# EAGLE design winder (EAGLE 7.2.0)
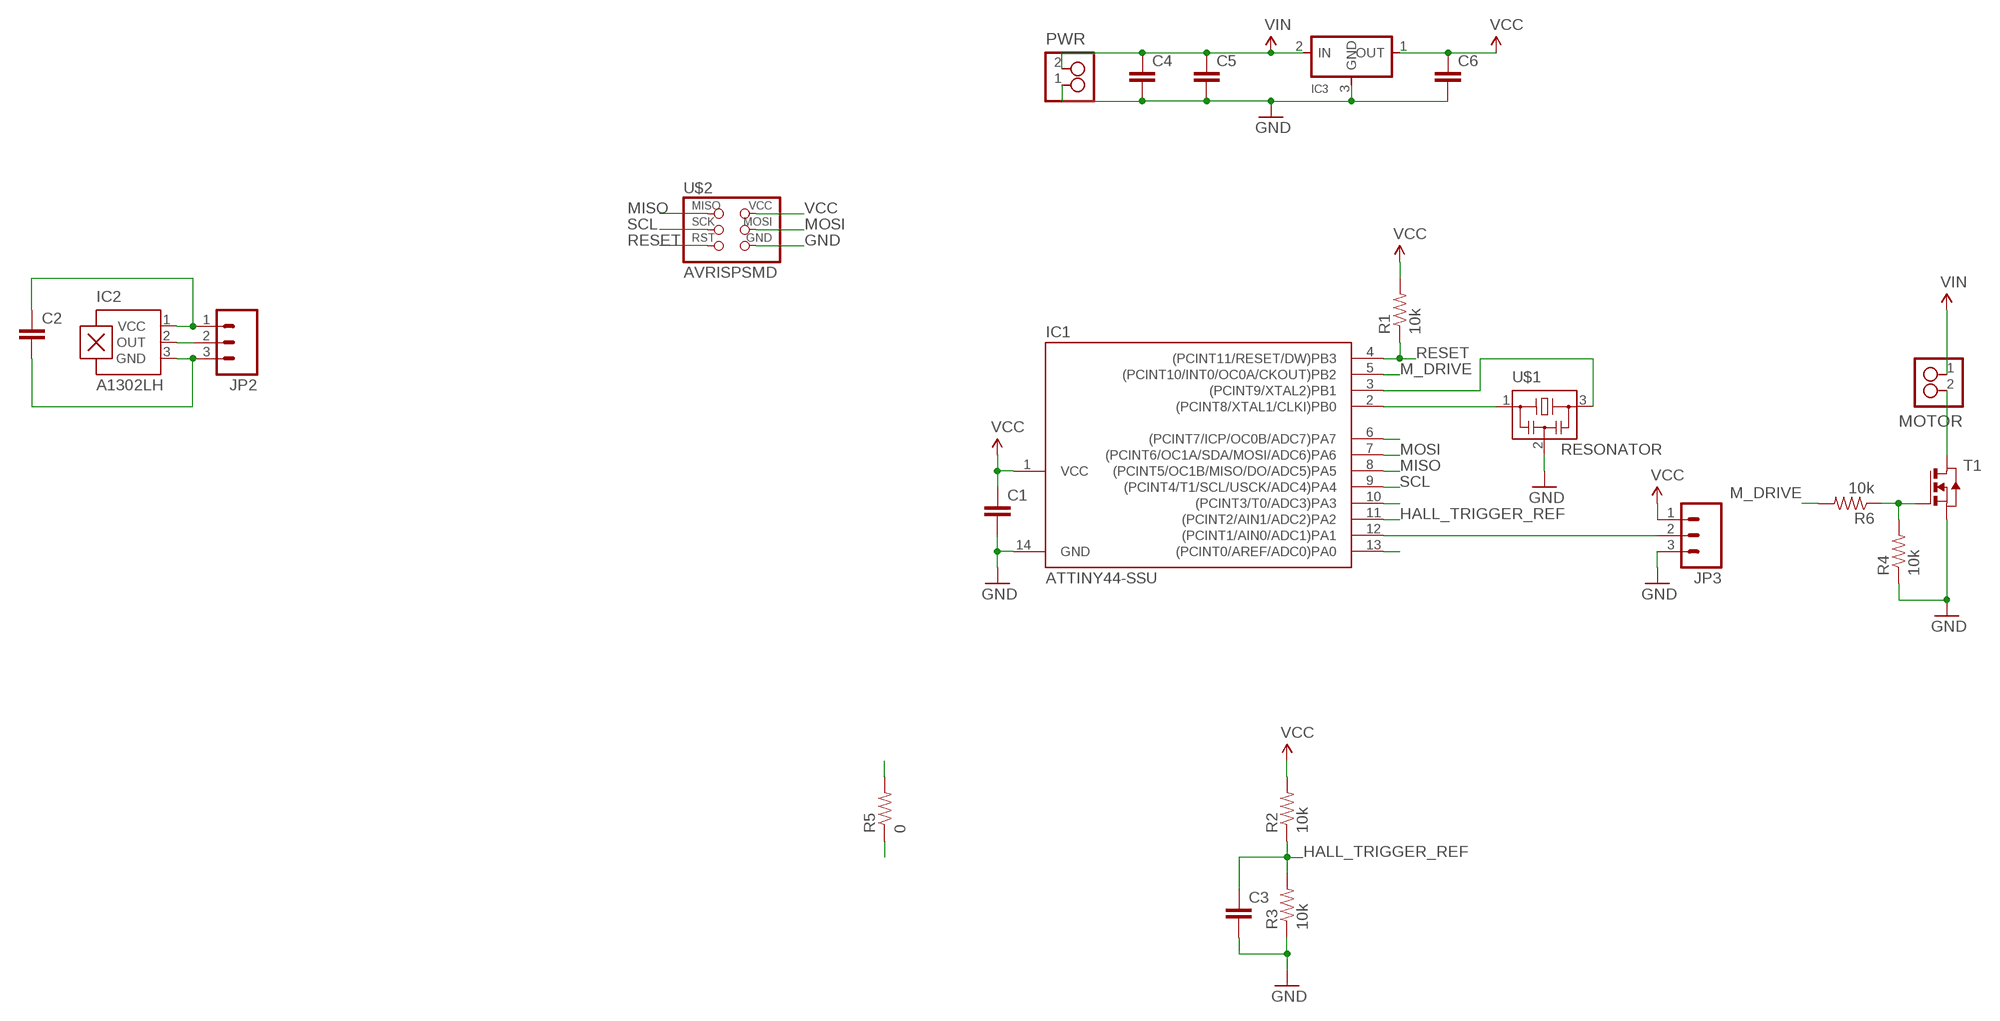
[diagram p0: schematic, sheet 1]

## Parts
C1  CAP1206  [1206]
C2  CAP1206  [1206]
C3  CAP1206  [1206]
C4  CAP1206  [1206]
C5  CAP1206  [1206]
C6  CAP1206  [1206]
IC1  ATTINY44-SSU  [SOIC14]
IC2  A1302LH  [SOT23-W]
IC3  REGULATORSOT23  [SOT23]
JP2  M03SMD_RA_MALE  [1X03_SMD_RA_MALE]
JP3  M03SMD_RA_MALE  [1X03_SMD_RA_MALE]
MOTOR  2_PIN_HEADERSCREW  [SCREW_2]
PWR  2_PIN_HEADERSCREW  [SCREW_2]
R1  10k  RESISTOR1206  [1206]
R2  10k  RESISTOR1206  [1206]
R3  10k  RESISTOR1206  [1206]
R4  10k  RESISTOR1206  [1206]
R5  0  RESISTOR1206  [1206]
R6  10k  RESISTOR1206  [1206]
T1  NMOSFETSOT23  [SOT-23]
U$1  RESONATOR  [EFOBM]
U$2  AVRISPSMD  [2X03SMD]

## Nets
GATE: R4.2 R6.1 T1.3(G)
GND: C1.2 C3.2 C4.2 C5.2 C6.2 IC1.14(GND) IC3.3(GND) JP3.3 PWR.1 R3.1 R4.1 T1.2(S) U$1.2 U$2.6(GND)
HALL_TRIGGER_REF: C3.1 IC1.11((PCINT2/AIN1/ADC2)PA2) R2.1 R3.2
M_DRIVE: IC1.5((PCINT10/INT0/OC0A/CKOUT)PB2) R6.2
MISO: IC1.8((PCINT5/OC1B/MISO/DO/ADC5)PA5) U$2.1(MISO)
MOSI: IC1.7((PCINT6/OC1A/SDA/MOSI/ADC6)PA6) U$2.4(MOSI)
N$1: C2.1 IC2.1(VCC) JP2.1
N$2: IC2.2(OUT) JP2.2
N$3: C2.2 IC2.3(GND) JP2.3
N$4: MOTOR.2 T1.1(D)
N$6: IC1.3((PCINT9/XTAL2)PB1) U$1.3
N$7: IC1.2((PCINT8/XTAL1/CLKI)PB0) U$1.1
N$8: IC1.6((PCINT7/ICP/OC0B/ADC7)PA7)
N$12: IC1.10((PCINT3/T0/ADC3)PA3)
N$14: IC1.12((PCINT1/AIN0/ADC1)PA1) JP3.2
N$15: IC1.13((PCINT0/AREF/ADC0)PA0)
RESET: IC1.4((PCINT11/RESET/DW)PB3) R1.1 U$2.5(RST)
SCL: IC1.9((PCINT4/T1/SCL/USCK/ADC4)PA4) U$2.3(SCK)
VCC: C1.1 C6.1 IC1.1(VCC) IC3.1(OUT) JP3.1 R1.2 R2.2 R5.1 R5.2 U$2.2(VCC)
VIN: C4.1 C5.1 IC3.2(IN) MOTOR.1 PWR.2

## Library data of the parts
C1-C6 = SparkFun-Passives:CAP: Capacitor
IC1 = fab:ATTINY44
IC2 = allegro:A13*?: Linear Hall Effect Sensor ICs Continuous-Time Ratiometric High-Temperature Operation Programmable Linear with Analog Output A1302 -Replacement- UGN3503 Source: http://www.allegromicro.com/en/Products/Part_Numbers/1301/1301.pdf http://www.allegromicro.com/en/Products/Part_Numbers/1321/1321.pdf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; MF: ALLEGRO MICROSYSTEMS, INC.; MPN: A1302ELHLT-T; OC_FARNELL: 1457209; OC_NEWARK: 31K6638
IC3 = fab:REGULATOR
JP2 JP3 = SparkFun-Connectors:M03: Header 3 Standard 3-pin 0.1" header. Use with straight break away headers (SKU : PRT-00116), right angle break away headers (PRT-00553), swiss pins (PRT-00743), machine pins (PRT-00117), and female headers (PRT-00115). Molex polarized connector foot print use with SKU : PRT-08232 with associated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; PROD_ID: CONN-10925
MOTOR PWR = ng:2_PIN_HEADER: 2 SMT pin pads
R1-R6 = SparkFun-Passives:RESISTOR: Resistor
T1 = ng:NMOSFET: MOS FET
U$1 = fab:RESONATOR
U$2 = fab:AVRISP

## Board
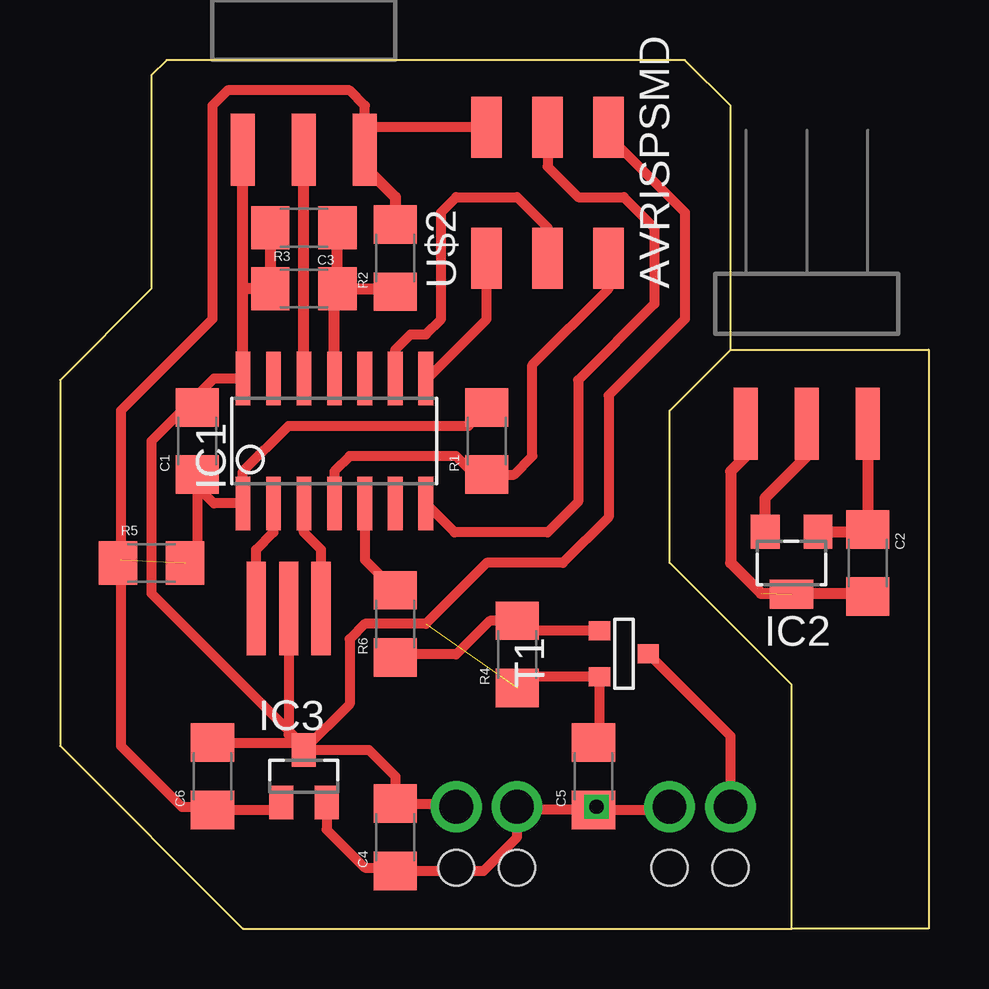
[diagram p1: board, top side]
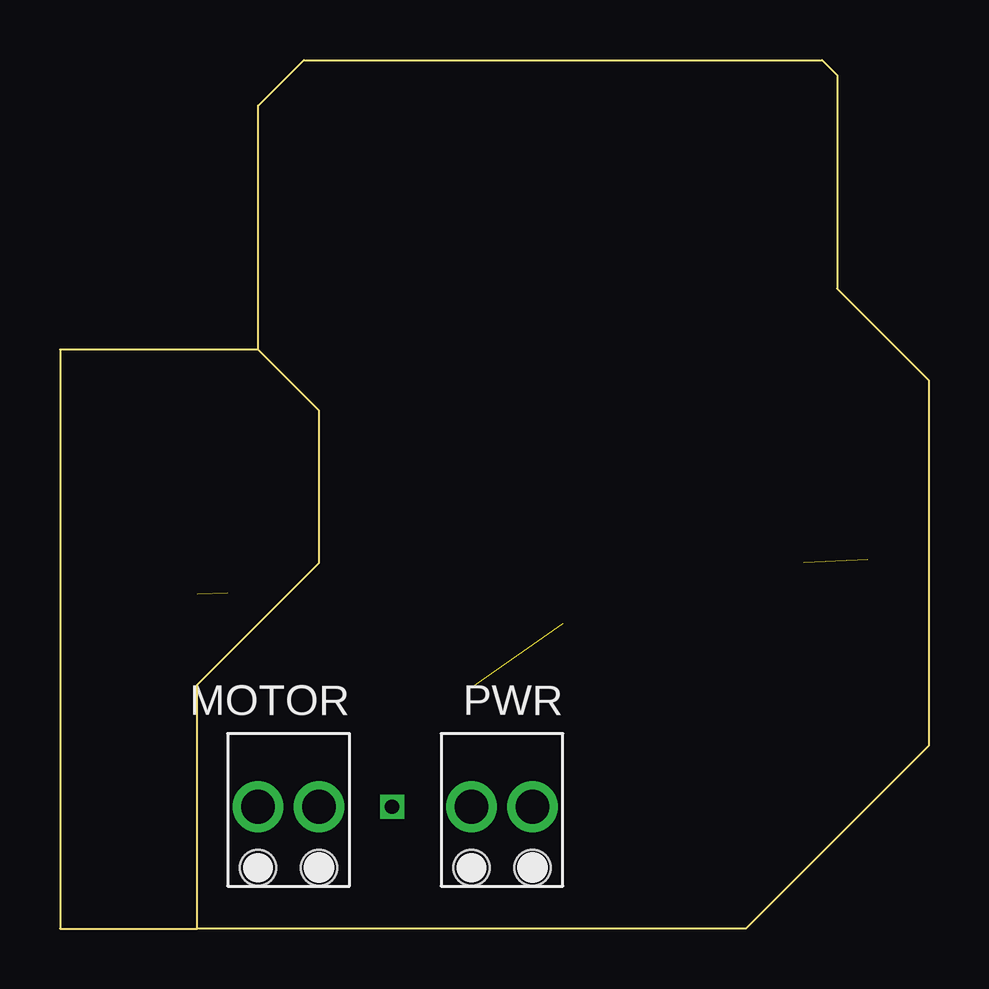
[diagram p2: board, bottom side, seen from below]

Size 36.2 x 36.19 mm. Coordinates in mm from the lower left corner, seen from the top.
Outline: 30.48,0 7.62,0 0,7.62 0,22.86 3.81,26.67 3.81,35.56 4.45,36.19 26.03,36.19 27.94,34.29 27.94,24.13
Outline: 30.48,0 30.48,10.16 25.4,15.24 25.4,21.59 27.94,24.13
Outline: 27.94,24.13 36.2,24.13 36.2,0 30.48,0
Copper layers (1*16): Top 0.035mm / dielectric 1.5mm / Bottom 0.035mm
Design rules "default": minimum track width 10mil, minimum drill 24mil, track to track 8mil, track to pad 8mil, pad to pad 8mil, via to via 8mil, smd to smd 8mil, copper to edge 40mil, drill to drill 8mil, minimum pad ring 10mil, minimum via ring 8mil, stop-mask expansion 4mil, vias tented up to drill 0mil, thermal gap 10mil

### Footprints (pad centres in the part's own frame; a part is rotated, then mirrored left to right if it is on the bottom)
1206 = smd 1.6 x 1.8: 1 -1.4,0; 2 1.4,0
SOIC14 = smd 0.61 x 2.21: 1 -3.81,-2.603; 2 -2.54,-2.603; 3 -1.27,-2.603; 4 0,-2.603; 5 1.27,-2.603; 6 2.54,-2.603; 7 3.81,-2.603; 8 3.81,2.603; 9 2.54,2.603; 10 1.27,2.603; 11 0,2.603; 12 -1.27,2.603; 13 -2.54,2.603; 14 -3.81,2.603
SOT23-W = smd 1.2 x 1.4: 1 -1.1,-1.3; 2 1.1,-1.3 | smd 1.8 x 1.2: 3 0,1.3
SOT23 = smd 1 x 1.4: 1 -0.95,-1.1; 2 0.95,-1.1; 3 0,1.1
1X03_SMD_RA_MALE = smd 1 x 3: 1 -2.54,5; 2 0,5; 3 2.54,5
SCREW_2 = drill 1.4 pad 2.108: 1 -1.27,-1.27; 2 1.27,-1.27 | hole 1.5: 1.27,1.27; -1.27,1.27
SOT-23 = smd 0.787 x 0.889: 1 0.025,-1.016; 2 -0.94,1.016; 3 0.991,1.016
EFOBM = smd 0.8 x 3.9: 1 -1.35,0; 2 0,0; 3 1.35,0
2X03SMD = smd 2.54 x 1.27: 1 -2.54,2.54; 2 2.92,2.54; 3 -2.54,0; 4 2.92,0; 5 -2.54,-2.54; 6 2.92,-2.54

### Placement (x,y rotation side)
C1  5.72,20.32 90 top
C2  33.66,15.24 270 top
C3  10.16,29.21 180 top
C4  13.97,3.81 90 top
C5  22.22,6.35 90 top
C6  6.35,6.35 90 top
IC1  11.43,20.32 0 top
IC2  30.48,15.24 180 top
IC3  10.16,6.35 0 top
JP2  31.11,26.04 180 top
JP3  10.16,37.47 180 top
MOTOR  26.67,3.81 180 bottom
PWR  17.78,3.81 180 bottom
R1  17.78,20.32 90 top
R2  13.97,27.94 90 top
R3  10.16,26.67 0 top
R4  19.05,11.43 90 top
R5  3.81,15.24 0 top
R6  13.97,12.7 90 top
T1  23.5,11.43 90 top
U$1  9.52,13.33 0 top
U$2  20.32,30.48 90 top

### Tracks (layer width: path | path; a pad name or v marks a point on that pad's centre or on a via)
GATE
  Top 0.406: T1.3 19.46,12.42 R4.2 17.91,12.83 16.51,11.43 14.1,11.43 R6.1
GND  (1 unrouted)
  Top 0.406: IC1.14 6.41,22.92 5.72,22.22 C1.2 5.21,21.72 3.81,20.32 3.81,13.97 9.86,7.92 9.86,7.75 | IC3.3 12.87,7.45 13.97,6.35 C4.2 | 13.97,5.08 C4.2 | C6.2 9.86,7.75 | 9.86,7.75 IC3.3 | R4.1 19.51,10.49 T1.2 22.48,8 C5.2 | U$1.2 9.52,8.09 IC3.3 | U$2.6 22.86,33.02 26.03,29.85 26.03,25.4 22.86,22.22 22.86,17.14 20.95,15.24 17.78,15.24 15.24,12.7 12.7,12.7 12.06,12.07 12.06,9.36 IC3.3 | C4.2 16.38,5.21 PWR.1
  Top 0.457: IC1.14 7.62,26.67 | 7.62,26.67 JP3.3 | C3.2 R3.1 7.62,26.67
HALL_TRIGGER_REF
  Top 0.457: R3.2 13.84,26.67 R2.1 | IC1.11 11.43,26.54 R3.2 | R3.2 C3.1
M_DRIVE
  Top 0.406: IC1.5 12.7,15.37 R6.2
MISO
  Top 0.406: 15.3,22.86 IC1.8 15.3,22.92 17.78,25.4 U$2.1
MOSI
  Top 0.406: U$2.4 20.32,31.75 21.59,30.48 23.5,30.48 24.77,29.21 24.77,26.04 21.59,22.86 21.59,17.78 20.32,16.51 16.45,16.51 IC1.7
N$1
  Top 0.457: JP2.1 C2.1 33.56,16.54 IC2.1
N$2
  Top 0.457: IC2.2 29.38,17.95 31.11,19.68 JP2.2
N$3  (1 unrouted)
  Top 0.457: JP2.3 28.58,19.68 27.94,19.05 27.94,15.24 29.21,13.97 33.53,13.97 C2.2
N$4
  Top 0.406: MOTOR.2 27.94,8.03 T1.1
N$6
  Top 0.406: IC1.3 10.16,16.51 10.88,15.79 U$1.3
N$7
  Top 0.406: U$1.1 8.18,15.79 8.89,16.51 IC1.2
N$14
  Top 0.457: IC1.12 JP3.2
RESET
  Top 0.406: IC1.4 11.43,19.05 12.06,19.68 16.51,19.68 17.27,18.92 R1.1 18.92,18.92 19.69,19.68 19.69,23.5 22.86,26.67 U$2.5
SCL
  Top 0.406: IC1.9 13.97,24.13 14.61,24.76 15.24,24.76 15.88,25.4 15.88,29.85 16.51,30.48 19.05,30.48 20.32,29.21 U$2.3
VCC  (1 unrouted)
  Top 0.406: 5.72,18.42 6.41,17.72 IC1.1 7.62,19.05 9.52,20.96 17.02,20.96 R1.2 | 5.72,18.42 C1.1 | 5.72,18.42 5.72,15.75 R5.2 | 12.7,31.75 12.7,33.02 | 12.7,33.02 12.7,34.29 12.06,34.92 6.98,34.92 6.35,34.29 6.35,25.4 2.54,21.59 2.54,15.37 | 2.54,15.37 R5.1 | U$2.2 13.08,33.4 12.7,33.02 | IC3.1 8.91,4.95 C6.1 6.22,5.08 5.08,5.08 2.54,7.62 2.54,15.37
  Top 0.457: JP3.1 12.7,31.75 13.97,30.48 R2.2
VIN  (via drill 0.6)
  Top 0.406: v22.36,5.08 C5.1 | IC3.2 11.11,4.13 12.7,2.54 13.84,2.54 C4.1 17.65,2.41 19.05,3.81 PWR.2 19.18,4.95 C5.1 | C5.1 25.27,4.95 MOTOR.1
